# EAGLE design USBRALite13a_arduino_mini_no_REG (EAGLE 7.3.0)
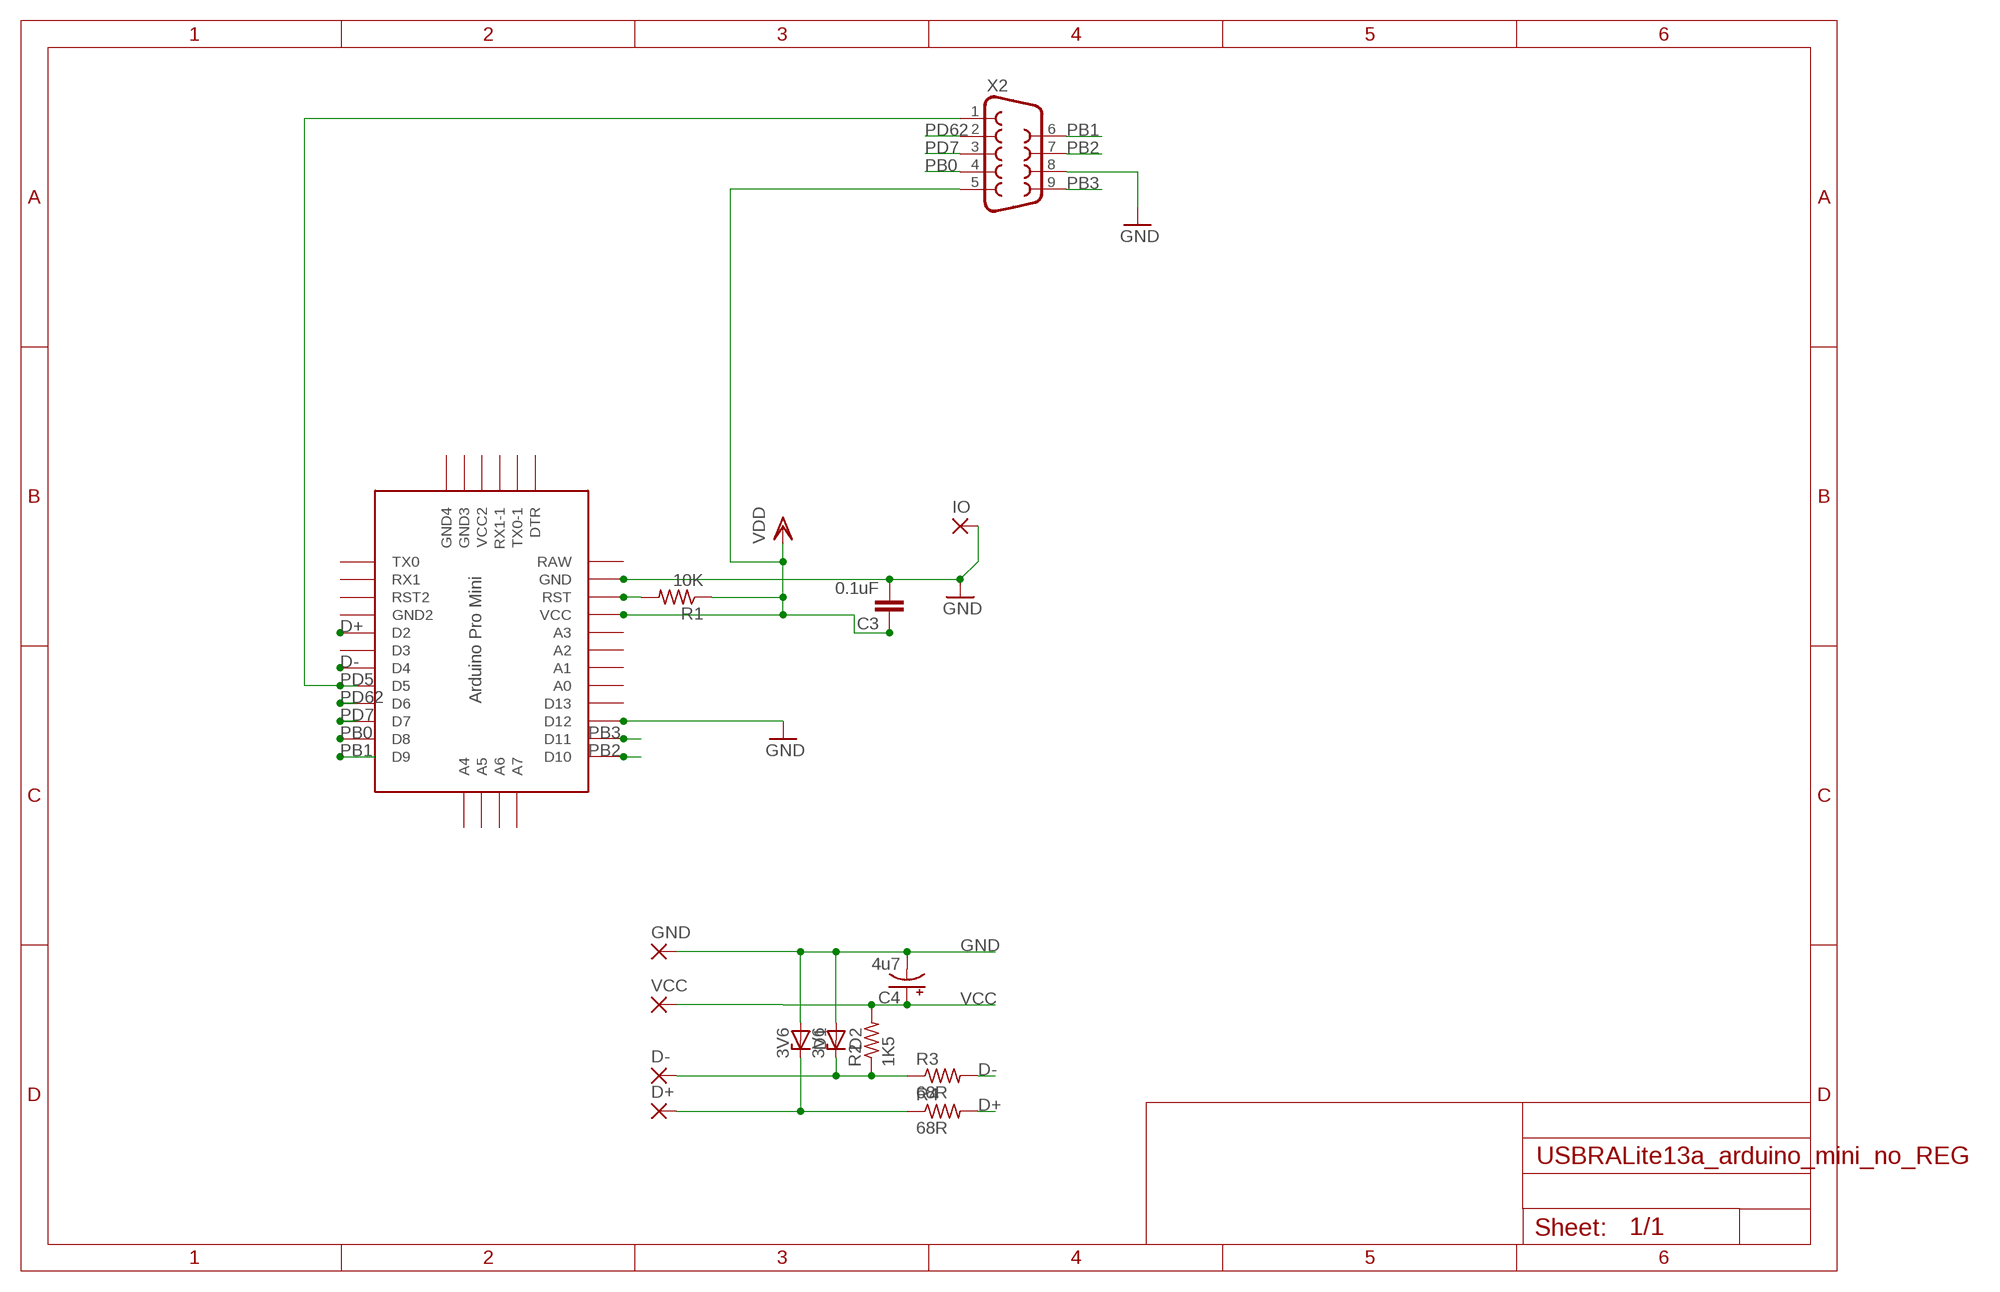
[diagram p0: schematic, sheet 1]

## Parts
C3  0.1uF  C-EU050-024X044  [C050-024X044]
C4  4u7  CPOL-USE2.5-6  [E2,5-6]
D1  3V6  ZENER-DIODEZD-5  [ZDIO-5]
D2  3V6  ZENER-DIODEZD-5  [ZDIO-5]
D+  1,6/0,9  [1,6/0,9]
D-  1,6/0,9  [1,6/0,9]
GND  1,6/0,9  [1,6/0,9]
IO  1,6/0,9  [1,6/0,9]
R1  10K  R-US_0207/10  [0207/10]
R2  1K5  R-US_0207/10  [0207/10]
R3  68R  R-US_0207/10  [0207/10]
R4  68R  R-US_0207/10  [0207/10]
U$1  PRO-MINI  [PRO-MINI]
VCC  1,6/0,9  [1,6/0,9]
X2  DB9MALE  [DB9_MALE]

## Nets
D+: R4.2 U$1.D2
D-: R3.2 U$1.D4
GND: C3.2 C4.- D1.A D2.A GND.1(P) IO.1(P) U$1.D12 U$1.GND X2.8
N$1: R1.2 U$1.RST
N$2: D2.C D-.1(P) R2.1 R3.1
N$8: D1.C D+.1(P) R4.1
PB0: U$1.D8 X2.4
PB1: U$1.D9 X2.6
PB2: U$1.D10 X2.7
PB3: U$1.D11 X2.9
PD5: U$1.D5 X2.1
PD7: U$1.D7 X2.3
PD62: U$1.D6 X2.2
VCC: C3.1 C4.+ R1.1 R2.2 U$1.VCC VCC.1(P) X2.5 ; supply symbol labelled VDD
Unconnected: U$1.A0 U$1.A1 U$1.A2 U$1.A3 U$1.A4 U$1.A5 U$1.A6 U$1.A7 U$1.D3 U$1.D13 U$1.DTR U$1.GND1(GND2) U$1.GND2(GND4) U$1.GND3 U$1.RST1(RST2) U$1.RX1 U$1.RX1-1 U$1.TX0 U$1.TX0-1 U$1.VCC1(VCC2)

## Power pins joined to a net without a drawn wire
RAW: U$1.RAW

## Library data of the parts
C3 = rcl:C-EU: CAPACITOR, European symbol
C4 = adafruit:CPOL-US: POLARIZED CAPACITOR, American symbol
D1 D2 = diode:ZENER-DIODE: Z-Diode
D+ D- GND IO VCC = wirepad:1,6/0,9: THROUGH-HOLE PAD
R1-R4 = adafruit:R-US_: RESISTOR, American symbol
U$1 = Arduino-clone:PRO-MINI: Arduion Pro Mini Clone V1.0 www.betemcu.cu
X2 = SparkFun:DB9: DB9 Connector Standard DB9 (D-Sub 9) serial connector. Can be used for CAN bus as well as RS485 and RS232. Footprint production proven. Spark Fun Electronics SKU : PRT-00429

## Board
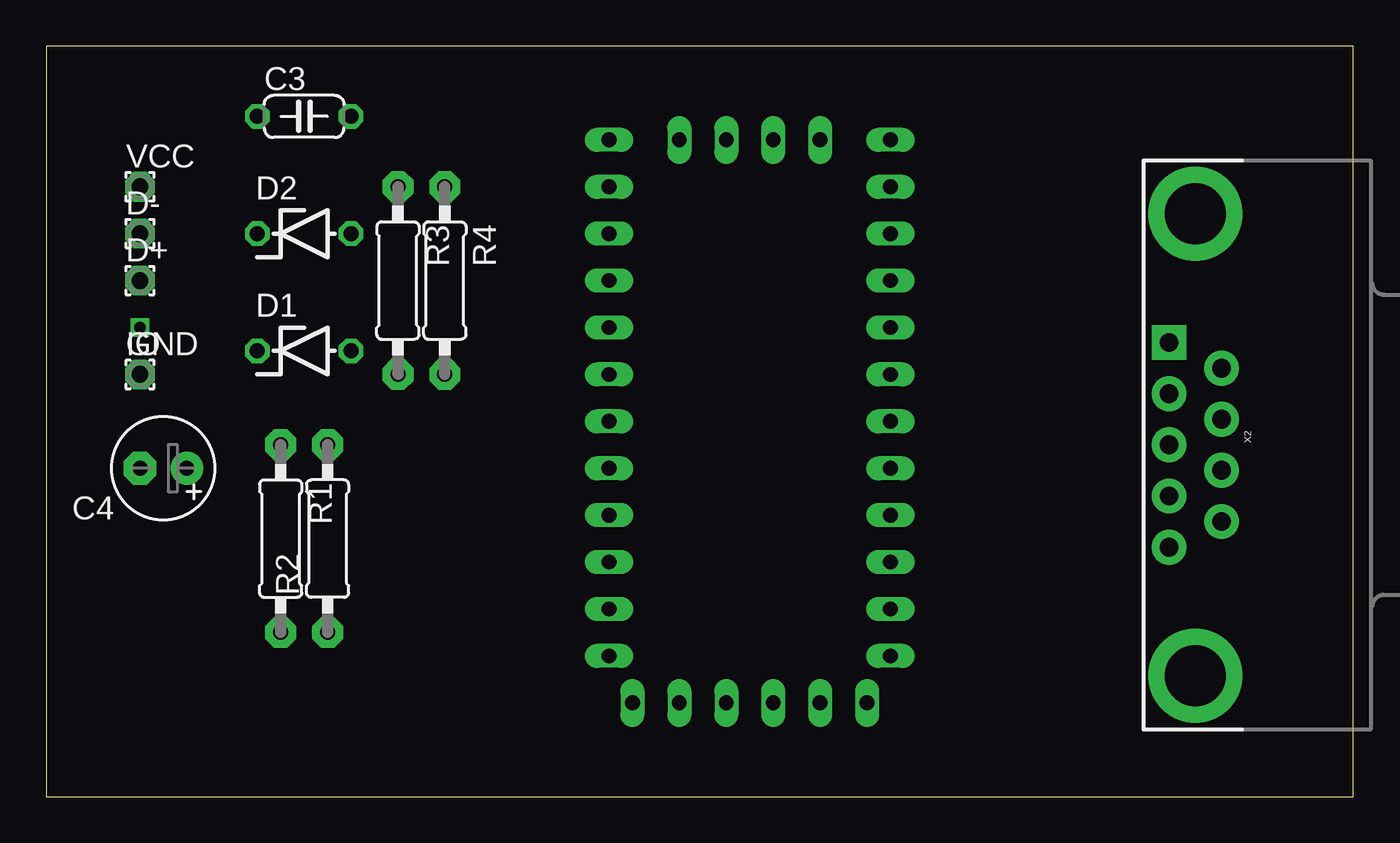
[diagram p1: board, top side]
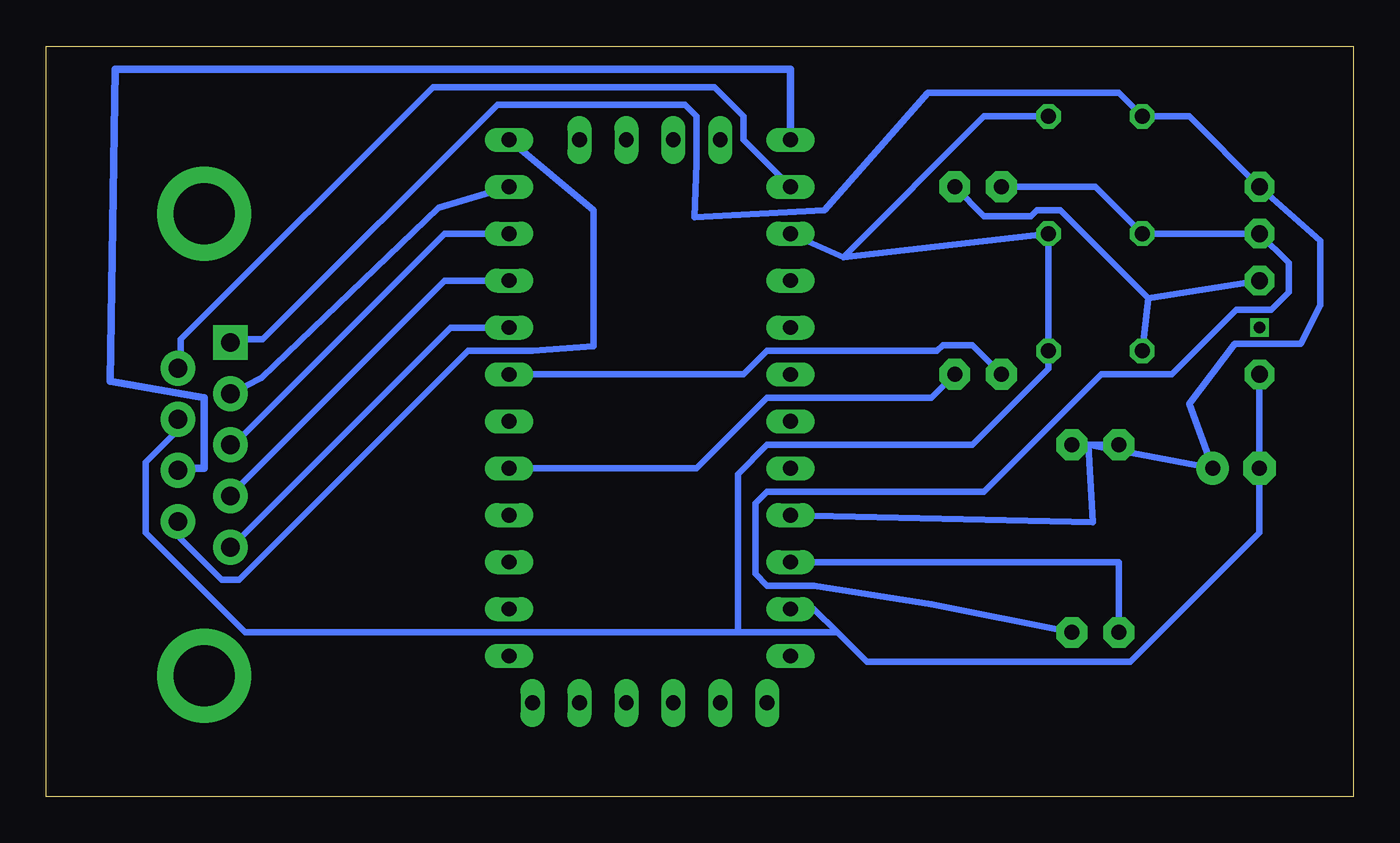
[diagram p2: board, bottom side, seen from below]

Size 70.79 x 40.63 mm. Coordinates in mm from the lower left corner, seen from the top.
Outline: 0,0 70.79,0 70.79,40.63 0,40.63 0,0
Copper layers (1*16): Top 0.035mm / dielectric 1.5mm / Bottom 0.035mm
Design rules "default *": minimum track width 14mil, minimum drill 24mil, track to track 16mil, track to pad 16mil, pad to pad 16mil, via to via 16mil, smd to smd 16mil, copper to edge 40mil, drill to drill 8mil, minimum pad ring 10mil, minimum via ring 8mil, stop-mask expansion 4mil, vias tented up to drill 0mil, thermal gap 10mil

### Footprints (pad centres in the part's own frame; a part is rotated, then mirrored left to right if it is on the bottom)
C050-024X044 = drill 0.813 octagon: 1 -2.54,0; 2 2.54,0
E2,5-6 = drill 0.813 pad 1.778: + -1.27,0 | drill 0.813 pad 1.778 octagon: - 1.27,0
ZDIO-5 = drill 0.813 octagon: A 2.54,0; C -2.54,0
1,6/0,9 = drill 0.914 pad 1.6 octagon: 1 0,0
0207/10 = drill 0.813 pad 1.676 octagon: 1 -5.08,0; 2 5.08,0
PRO-MINI = drill 0.8 long: A0 8.89,8.89; A1 8.89,11.43; A2 8.89,13.97; A3 8.89,16.51; A4 -2.54,-1.27; A5 0,-1.27; A6 2.54,-1.27; A7 5.08,-1.27; D2 -6.35,16.51; D3 -6.35,13.97; D4 -6.35,11.43; D5 -6.35,8.89; D6 -6.35,6.35; D7 -6.35,3.81; D8 -6.35,1.27; D9 -6.35,-1.27; D10 8.89,-1.27; D11 8.89,1.27; D12 8.89,3.81; D13 8.89,6.35; DTR 7.62,29.21; GND 8.89,24.13; GND1 -6.35,19.05; GND2 -5.08,29.21; GND3 -2.54,29.21; RAW 8.89,26.67; RST 8.89,21.59; RST1 -6.35,21.59; RX1 -6.35,24.13; RX1-1 2.54,29.21; TX0 -6.35,26.67; TX0-1 5.08,29.21; VCC 8.89,19.05; VCC1 0,29.21
DB9_MALE = drill 1.016 pad 1.88: 1 5.54,-1.42; 2 2.77,-1.42; 3 0,-1.42; 4 -2.77,-1.42; 6 4.15,1.42; 7 1.38,1.42; 8 -1.38,1.42; 9 -4.15,1.42 | drill 1.016 pad 1.88 square: 5 -5.54,-1.42 | drill 3.302 pad 5.08: G1 -12.5,0; G2 12.5,0

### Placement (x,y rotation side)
C3  13.97,36.83 0 top
C4  6.35,17.78 180 top
D1  13.97,24.13 0 top
D2  13.97,30.48 0 top
D+  5.08,27.94 0 top
D-  5.08,30.48 0 top
GND  5.08,22.86 0 top
IO  5.08,22.86 0 top
R1  12.7,13.97 270 top
R2  15.24,13.97 90 top
R3  19.05,27.94 270 top
R4  21.59,27.94 270 top
U$1  39.37,34.29 180 top
VCC  5.08,33.02 0 top
X2  62.23,19.05 270 top

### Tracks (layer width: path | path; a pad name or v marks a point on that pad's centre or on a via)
D+
  Bottom 0.356: U$1.D2 35.56,17.78 31.75,21.59 22.86,21.59 R4.2
D-
  Bottom 0.356: U$1.D4 33.02,22.86 31.75,24.13 22.54,24.13 22.23,24.45 20.64,24.45 R3.2
GND
  Bottom 0.356: 27.62,29.21 D2.A D1.A 16.51,23.18 20.64,19.05 31.75,19.05 33.34,17.46 33.34,8.89 | 27.62,29.21 U$1.D12 | C3.2 20,36.83 27.62,29.21 | U$1.GND 29.21,10.16 27.94,8.89 | 27.94,8.89 26.35,7.3 12.06,7.3 5.08,14.29 C4.- IO.1 | 27.94,8.89 33.34,8.89 | 33.34,8.89 60.01,8.89 65.41,14.29 65.41,18.1 63.82,19.69 63.82,20.32 X2.8
N$1
  Bottom 0.356: U$1.RST 12.7,12.7 R1.2
N$2
  Bottom 0.356: R2.1 22.86,10.41 29.21,11.43 31.75,11.43 32.38,12.07 32.38,15.88 31.75,16.51 20,16.51 13.65,22.86 9.84,22.86 6.35,26.35 4.45,26.35 3.49,27.3 3.49,28.89 D-.1 D2.C 13.97,33.02 R3.1
N$3  (via drill 0.6)
  other vias: 5.08,25.4
N$8
  Bottom 0.356: 11.11,26.99 D1.C | D+.1 11.11,26.99 | R4.1 20,31.43 17.46,31.43 17.14,31.75 15.88,31.75 11.11,26.99
PB0
  Bottom 0.356: U$1.D8 49.53,31.88 59.12,22.67 X2.4
PB1
  Bottom 0.356: U$1.D9 41.15,31.75 41.15,24.38 44.45,24.13 47.94,24.13 60.33,11.75 61.28,11.75 63.5,13.97 63.5,14.61 X2.6
PB2
  Bottom 0.406: U$1.D10 30.48,39.37 67.06,39.37 67.31,22.48 62.23,21.59 62.23,17.78 63.65,17.78 X2.7
PB3
  Bottom 0.356: U$1.D11 33.02,35.56 33.02,36.83 34.61,38.42 49.85,38.42 63.5,24.77 63.5,23.5 X2.9
PD5
  Bottom 0.356: U$1.D5 48.9,25.4 60.64,13.65 X2.1
PD7
  Bottom 0.356: U$1.D7 49.21,30.48 60.64,19.05 X2.3
PD62
  Bottom 0.356: U$1.D6 49.21,27.94 60.64,16.51 X2.2
VCC
  Bottom 0.356: U$1.VCC 14.1,14.86 14.35,19.05 | R2.2 14.35,19.05 | 14.35,19.05 R1.1 | 14.35,19.05 C4.+ 8.89,21.27 6.41,24.51 2.86,24.51 1.78,26.61 1.78,30.1 VCC.1 8.89,36.83 C3.1 12.7,38.1 23.05,38.1 28.64,31.75 35.69,31.37 35.56,34.29 35.56,36.83 36.2,37.46 46.35,37.46 59.05,24.77 60.64,24.77 X2.5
